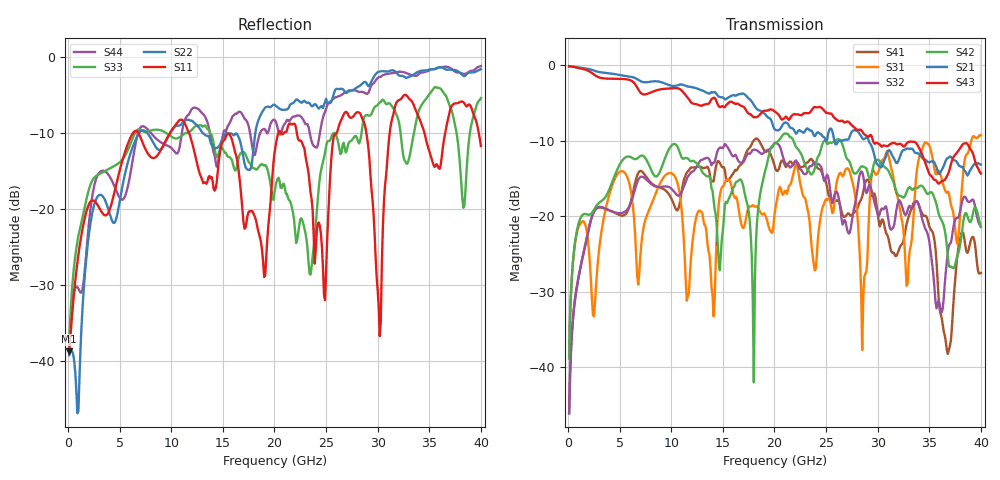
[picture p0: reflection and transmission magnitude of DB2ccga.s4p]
! ADC12DJ3200QML-SP
! 196-pin NWE package
! CCGA Ceramic Package with columns (ceramic column grid array)
! Texas Instruments 4/21/2021
! Single-ended  S-parameters
! PORT#  PORT_NAME  NET_NAME
! PORT1:  DAxN.DIEBUMP DAxN
! PORT2:  DAxN.BGA  DAxN
! PORT3:  DAxP.DIEBUMP DAxP
! PORT4:  DAxP.BGA  DAxP
! Touchstone Ver. 1.0
! Number of ports is 4
# Hz	S	MA	R	50.000000
! SCATTERING PARAMETERS  :
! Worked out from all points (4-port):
!   400 points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, 100 MHz to 40 GHz, reference 50 ohm
!   strongest paths, dB at 100 MHz, 10.1 GHz, 20.1 GHz, 30.1 GHz, 40 GHz:
!     S43: -0.1, -3.0, -6.2, -10.4, -14.3
!     S21: -0.1, -2.7, -8.5, -13.3, -13.1
!     S42: -38.8, -10.5, -10.3, -12.5, -21.4
!     S32: -46.1, -16.4, -10.2, -19.9, -21.4
!     S31: -38.8, -14.3, -18.8, -14.0, -9.3
!     S41: -46.1, -17.9, -13.7, -20.6, -27.5
!   lowest |S11| = -38.8 dB at 100 MHz (marker M1), VSWR 1.02, Z = 51.1 + j0.196 ohm
!   |S11| at or under -10 dB: start of sweep to 6.292 GHz; 11.72 GHz to 20.38 GHz (8.652 GHz wide, 53.9 % of centre); 22.17 GHz to 26.03 GHz (3.861 GHz wide, 16 % of centre)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
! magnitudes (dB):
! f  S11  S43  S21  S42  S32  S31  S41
! 100 MHz  -38.8  -0.1  -0.1  -38.8  -46.1  -38.8  -46.1
! 7 GHz  -10.5  -3.6  -2.1  -12.0  -14.8  -25.3  -14.0
! 18 GHz  -20.7  -6.9  -5.2  -42.0  -11.1  -18.6  -9.9
! 20.9 GHz  -10.0  -7.1  -7.7  -9.1  -12.5  -17.0  -12.9
! 30.2 GHz  -36.8  -10.5  -13.4  -12.7  -19.7  -13.5  -21.3
! 31.8 GHz  -6.0  -10.4  -12.9  -16.7  -19.3  -16.8  -25.3
! 40 GHz  -11.7  -14.3  -13.1  -21.4  -21.4  -9.3  -27.5
